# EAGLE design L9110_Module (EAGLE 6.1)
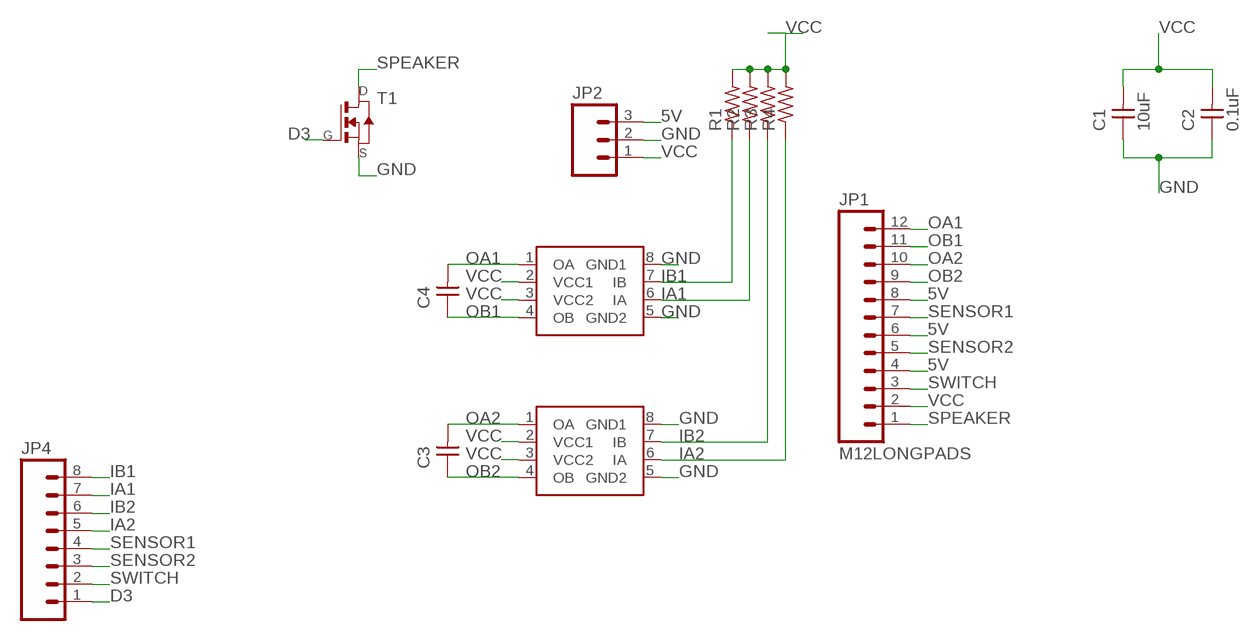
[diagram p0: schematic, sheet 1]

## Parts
C1  10uF  CAP-UNPOLARIZEDFAB  [C1206FAB]
C2  0.1uF  CAP-UNPOLARIZEDFAB  [C1206FAB]
C3  CAP-UNPOLARIZEDFAB  [C1206FAB]
C4  CAP-UNPOLARIZEDFAB  [C1206FAB]
JP1  M12LONGPADS  [1X12_LONGPADS]
JP2  M03LONGPADS  [1X03_LONGPADS]
JP4  M08LONGPADS  [1X08_LONGPADS]
R1  RES-US1206FAB  [R1206FAB]
R2  RES-US1206FAB  [R1206FAB]
R3  RES-US1206FAB  [R1206FAB]
R4  RES-US1206FAB  [R1206FAB]
T1  NMOSFETSOT23  [SOT-23]
U$1  L9110  L9110_SOP8  [SOIC8]
U$2  L9110_SOP8  [SOIC8]

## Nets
5V: JP1.4 JP1.6 JP1.8 JP2.3
D3: JP4.1 T1.3(G)
GND: C1.1 C2.1 JP2.2 T1.2(S) U$1.5(GND2) U$1.8(GND1) U$2.5(GND2) U$2.8(GND1)
IA1: JP4.7 R2.1 U$1.6(IA)
IA2: JP4.5 R4.1 U$2.6(IA)
IB1: JP4.8 R1.1 U$1.7(IB)
IB2: JP4.6 R3.1 U$2.7(IB)
OA1: C4.2 JP1.12 U$1.1(OA)
OA2: C3.2 JP1.10 U$2.1(OA)
OB1: C4.1 JP1.11 U$1.4(OB)
OB2: C3.1 JP1.9 U$2.4(OB)
SENSOR1: JP1.7 JP4.4
SENSOR2: JP1.5 JP4.3
SPEAKER: JP1.1 T1.1(D)
SWITCH: JP1.3 JP4.2
VCC: C1.2 C2.2 JP1.2 JP2.1 R1.2 R2.2 R3.2 R4.2 U$1.2(VCC1) U$1.3(VCC2) U$2.2(VCC1) U$2.3(VCC2)

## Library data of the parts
C1-C4 = fab:CAP-UNPOLARIZED
JP1 = SparkFun-Connectors:M12: Header 12 Standard 12-pin 0.1" header. Use with straight break away headers (SKU : PRT-00116), right angle break away headers (PRT-00553), swiss pins (PRT-00743), machine pins (PRT-00117), and female headers (PRT-00115).
JP2 = SparkFun-Connectors:M03: Header 3 Standard 3-pin 0.1" header. Use with straight break away headers (SKU : PRT-00116), right angle break away headers (PRT-00553), swiss pins (PRT-00743), machine pins (PRT-00117), and female headers (PRT-00115). Molex polarized connector foot print use with SKU : PRT-08232 with associated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
JP4 = SparkFun-Connectors:M08: Header 8 Standard 8-pin 0.1" header. Use with straight break away headers (SKU : PRT-00116), right angle break away headers (PRT-00553), swiss pins (PRT-00743), machine pins (PRT-00117), and female headers (PRT-00115).
R1-R4 = fab:RES-US: Resistor (US Symbol)
T1 = fab:NMOSFET: MOS FET
U$1 U$2 = fab:L9110_SOP8

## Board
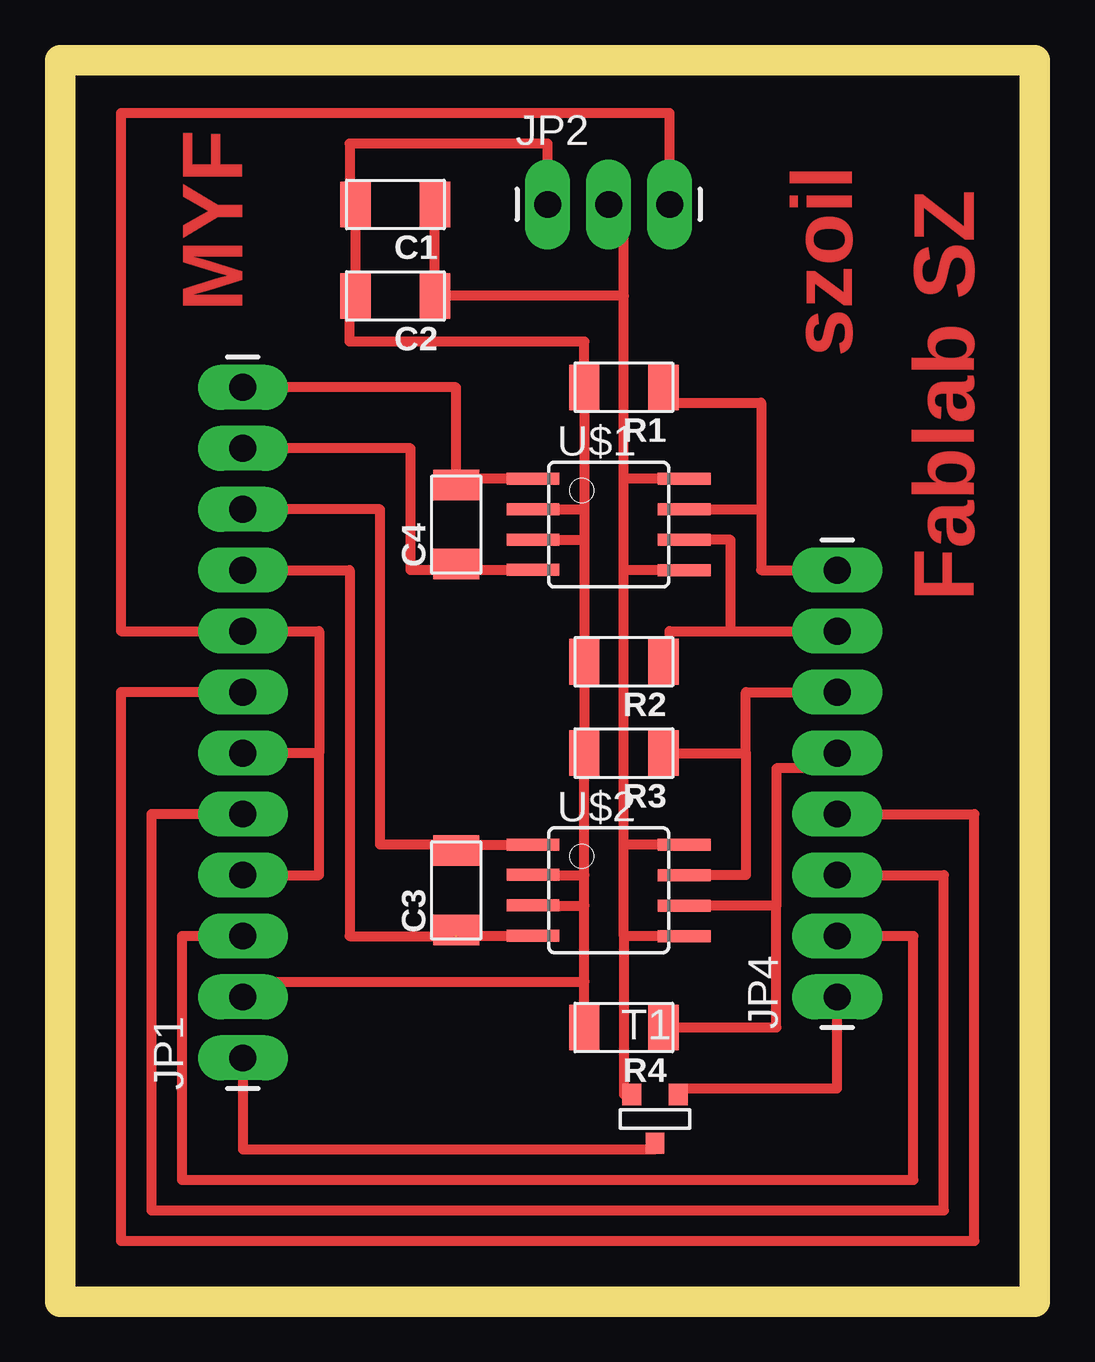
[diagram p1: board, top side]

Size 40.62 x 51.74 mm. Coordinates in mm from the lower left corner, seen from the top.
Outline: 0,0 40.62,0 40.62,51.74 0,51.74 0,0
Copper layers (1*16): Top 0.035mm / dielectric 1.5mm / Bottom 0.035mm
Design rules: minimum track width 10mil, minimum drill 24mil, track to track 8mil, track to pad 8mil, pad to pad 8mil, via to via 8mil, smd to smd 8mil, copper to edge 40mil, drill to drill 8mil, minimum pad ring 10mil, minimum via ring 8mil, stop-mask expansion 4mil, vias tented up to drill 0mil, thermal gap 10mil

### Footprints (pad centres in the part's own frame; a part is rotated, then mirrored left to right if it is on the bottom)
C1206FAB = smd 1.27 x 1.905: 1 -1.651,0; 2 1.651,0
1X12_LONGPADS = drill 1.118 pad 1.88 long: 1 0,0; 2 2.54,0; 3 5.08,0; 4 7.62,0; 5 10.16,0; 6 12.7,0; 7 15.24,0; 8 17.78,0; 9 20.32,0; 10 22.86,0; 11 25.4,0; 12 27.94,0
1X03_LONGPADS = drill 1.118 pad 1.88 long: 1 0,0; 2 2.54,0; 3 5.08,0
1X08_LONGPADS = drill 1.118 pad 1.88 long: 1 0,0; 2 2.54,0; 3 5.08,0; 4 7.62,0; 5 10.16,0; 6 12.7,0; 7 15.24,0; 8 17.78,0
R1206FAB = smd 1.27 x 1.905: 1 -1.651,0; 2 1.651,0
SOT-23 = smd 0.787 x 0.889: 1 0.025,-1.016; 2 -0.94,1.016; 3 0.991,1.016
SOIC8 = smd 0.5 x 2.2: 1 -1.905,-3.154; 2 -0.645,-3.154; 3 0.625,-3.154; 4 1.895,-3.154; 5 1.905,3.154; 6 0.635,3.154; 7 -0.635,3.154; 8 -1.905,3.154

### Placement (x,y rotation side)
C1  13.97,45.72 180 top
C2  13.97,41.91 180 top
C3  16.51,17.14 90 top
C4  16.51,32.38 90 top
JP1  7.62,10.16 90 top
JP2  20.32,45.72 0 top
JP4  32.38,12.7 90 top
R1  23.5,38.1 180 top
R2  23.5,26.67 180 top
R3  23.5,22.86 180 top
R4  23.5,11.43 180 top
T1  24.77,7.62 0 top
U$1  22.86,32.38 270 top
U$2  22.86,17.14 270 top

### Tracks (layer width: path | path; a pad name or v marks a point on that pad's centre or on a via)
5V
  Top 0.406: 10.79,22.86 10.79,27.94 JP1.8 2.54,27.94 2.54,49.53 25.4,49.53 JP2.3 | JP1.4 10.79,17.78 10.79,22.86 | 10.79,22.86 JP1.6
D3
  Top 0.406: T1.3 25.76,8.89 32.38,8.89 JP4.1
GND
  Top 0.406: U$2.8 23.5,19.05 | 23.5,19.05 23.5,30.48 | 23.5,30.48 23.5,34.29 | 23.5,15.24 23.5,19.05 | U$1.5 23.5,30.48 | U$1.8 23.5,34.29 | 23.5,34.29 23.5,41.91 | 23.5,41.91 C2.1 C1.1 | 23.5,41.91 23.5,45.72 JP2.2 | U$2.5 23.5,15.24 | 23.5,15.24 23.5,8.64 T1.2
IA1
  Top 0.406: R2.1 25.4,26.92 25.4,27.94 27.94,27.94 | 27.94,27.94 27.94,31.75 U$1.6 | 27.94,27.94 JP4.7
IA2
  Top 0.406: 29.84,16.51 29.84,22.23 31.75,22.23 31.75,22.86 JP4.5 | 29.84,16.51 U$2.6 | R4.1 29.84,11.43 29.84,16.51
IB1
  Top 0.406: U$1.7 29.21,33.02 | 29.21,33.02 29.21,30.48 JP4.8 | R1.1 25.15,37.46 29.21,37.46 29.21,33.02
IB2
  Top 0.406: R3.1 28.57,22.86 | 28.57,22.86 28.57,17.78 U$2.7 | 28.57,22.86 28.57,25.4 JP4.6
OA1
  Top 0.406: 16.51,34.29 C4.2 16.51,33.66 | 16.51,34.29 16.51,38.1 JP1.12 | U$1.1 16.51,34.29
OA2
  Top 0.406: 16.51,19.05 U$2.1 | C3.2 16.51,19.05 | 16.51,19.05 13.34,19.05 13.34,33.02 JP1.10
OB1
  Top 0.406: 16.51,30.48 14.61,30.48 14.61,35.56 JP1.11 | U$1.4 19.71,30.48 16.51,30.48 | 16.51,30.48 C4.1
OB2  (1 unrouted)
  Top 0.406: C3.1 16.51,15.25 U$2.4 | JP1.9 12.06,30.48 12.06,15.24 16.51,15.24
SENSOR1
  Top 0.406: JP1.7 2.54,25.4 2.54,2.54 38.1,2.54 38.1,20.32 JP4.4
SENSOR2
  Top 0.406: JP1.5 3.81,20.32 3.81,3.81 36.83,3.81 36.83,17.78 JP4.3
SPEAKER
  Top 0.406: JP1.1 7.62,6.35 24.77,6.35 24.77,6.6 T1.1
SWITCH
  Top 0.406: JP1.3 5.08,15.24 5.08,5.08 35.56,5.08 35.56,15.24 JP4.2
VCC
  Top 0.406: 21.84,33.02 R1.2 21.84,40 12.06,40 12.06,41.91 C2.2 C1.2 12.06,45.72 12.06,48.26 20.32,48.26 JP2.1 | 21.84,33.02 21.84,31.75 | 21.84,31.75 R2.2 R3.2 21.84,17.78 | R4.2 21.84,13.34 | 21.84,13.34 21.84,16.51 | 21.84,16.51 21.84,17.78 | U$2.2 19.72,17.78 21.84,17.78 | U$2.3 19.72,16.51 21.84,16.51 | U$1.3 19.72,31.75 21.84,31.75 | U$1.2 19.72,33.02 21.84,33.02 | JP1.2 7.62,13.34 21.84,13.34

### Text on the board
Top: MYF | szoil | Fablab SZ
